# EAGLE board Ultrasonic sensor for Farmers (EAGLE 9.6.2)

Size 205.11 x 164.31 mm. Coordinates in mm from the lower left corner, seen from the top.
Outline: 0,0 205.11,0 205.11,164.31 0,164.31 0,0
Copper layers (1*16): Top 0.035mm / dielectric 1.5mm / Bottom 0.035mm
Design rules "default": minimum track width 6mil, minimum drill 0.35mm, track to track 6mil, track to pad 6mil, pad to pad 6mil, via to via 6mil, smd to smd 6mil, copper to edge 40mil, drill to drill 6mil, minimum pad ring 10mil, minimum via ring 8mil, stop-mask expansion 4mil, vias tented up to drill 0mil, thermal gap 10mil

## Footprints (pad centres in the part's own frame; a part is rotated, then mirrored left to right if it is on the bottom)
HC-SR04 = drill 1.016 long: 1 -3.81,0; 2 -1.27,0; 3 1.27,0; 4 3.81,0
SG90 = drill 1.016 long: 1 -2.54,0; 2 0,0; 3 2.54,0
ARDUINO-UNO-R3-SHIELD = drill 1.016 pad 1.88: 3.3V 24.13,-2.54; 5V 24.13,0; A0 24.13,12.7; A1 24.13,15.24; A2 24.13,17.78; A3 24.13,20.32; A4 24.13,22.86; A5 24.13,25.4; AREF -24.13,-13.97; D2 -24.13,20.32; D3 -24.13,17.78; D4 -24.13,15.24; D5 -24.13,12.7; D6 -24.13,10.16; D7 -24.13,7.62; D8 -24.13,3.81; D9 -24.13,1.27; D10 -24.13,-1.27; D11 -24.13,-3.81; D12 -24.13,-6.35; D13 -24.13,-8.89; GND@0 24.13,2.54; GND@1 24.13,5.08; GND@2 -24.13,-11.43; IOREF 24.13,-7.62; NC 24.13,-10.16; RES 24.13,-5.08; RX -24.13,25.4; SCL -24.13,-19.05; SDA -24.13,-16.51; TX -24.13,22.86; VIN 24.13,7.62
LCD-I2C = drill 1.016 long: 1 -19.05,-5.08; 2 -19.05,-7.62; 3 -19.05,-10.16; 4 -19.05,-12.7

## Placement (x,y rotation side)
DIST1  DISTANCE-SENSOR-4PINHC-SR04  [HC-SR04]  123.12,110.45 0 top
SERVO1  SERVOSG90  [SG90]  174.27,157.33 180 top
U1  ARDUINO-UNO-R3-SHIELD  [ARDUINO-UNO-R3-SHIELD]  47.88,70.91 270 top
U2  LCD-16X2-I2CSUNFOUNDER-IIC  [LCD-I2C]  149.49,36.63 0 top

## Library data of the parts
DIST1 SERVO1 U1 U2 = Tinkercad

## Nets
U1_5V: DIST1.1 SERVO1.2 U1.5V U2.2
U1_D4: DIST1.3 U1.D4
U1_D5: DIST1.2 U1.D5
U1_D7: SERVO1.3 U1.D7
U1_GND: DIST1.4 SERVO1.1 U1.GND@0 U1.GND@1 U1.GND@2 U2.1
U1_SCL: U1.SCL U2.4
U1_SDA: U1.SDA U2.3

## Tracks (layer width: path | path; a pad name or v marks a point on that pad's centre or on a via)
U1_5V  (3 unrouted)
U1_D4  (1 unrouted)
U1_D5  (1 unrouted)
U1_D7  (1 unrouted)
U1_GND  (5 unrouted)
U1_SCL  (1 unrouted)
U1_SDA  (1 unrouted)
